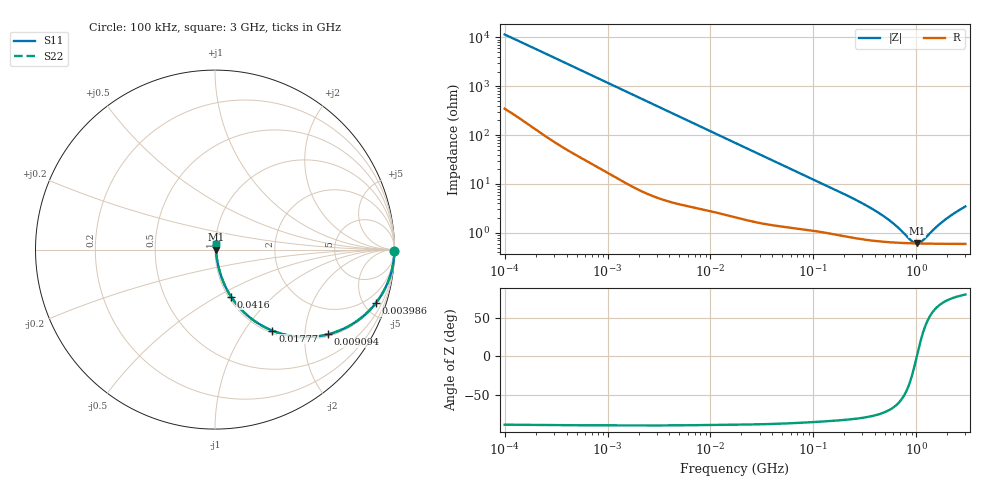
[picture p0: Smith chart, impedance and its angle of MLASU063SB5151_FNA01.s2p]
! MLASU063SB5151_FNA01  S-PARAMETER MODEL  ( Standard Model )
! Model Generated by TAIYO YUDEN Corporation (http://www.ty-top.com)
! Version 1.0
! TAIYO YUDEN Control No. 220601
! Copyright(c) 2012 TAIYO YUDEN CO.,LTD. All Rights Reserved.
! Product Description (link to TY-COMPAS)
! https://ds.yuden.co.jp/TYCOMPAS/or/detail?pn=MLASU063SB5151KFNA01&u=M
! Products Name : Multilayer Ceramic Capacitors
! Characteristics :
!  Capacitance : 150 [pF] , Rated Voltage : 50 [V] , TCC : B / X5R
!  Case Size : 0.6 x 0.3 / 0.024 x 0.012 [mm/inch] , Thickness : 0.3 / 0.012 [mm/inch]
!  (Conditions: Temperature = 25 [degC] , DC Bias Voltage = 0 [V])
! External Node Assignments :
!  1  o---| |---o  2
! GND o---------o GND
! Frequency Range : 100kHz  -  3GHz  [ 401 STEP ]
# MHZ S RI R 50
! Freq[MHz].  S11 Real  S11 Imag  S21 Real  S21 Imag  S12 Real  S12 Imag  S22 Real  S22 Imag
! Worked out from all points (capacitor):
!   401 points, 100 kHz to 3 GHz, reference 50 ohm
!   read as one part in series: C = 138 pF near 105.3 kHz
!   lowest |Z| = 606 mohm at 1.016 GHz (marker M1)
!   series resonance near 1.012 GHz, so ESL is about 180 pH
!   S11 on the Smith chart (normalised r, x): 100 kHz: open; 3.986 MHz: 1.09, -5.96; 9.094 MHz: 1.06, -2.63; 17.77 MHz: 1.04, -1.36; 41.6 MHz: 1.03, -0.58; 3 GHz: 1.01, +0.07
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0.1  0.9997 -0.00871  0.000339 0.00871  0.000339 0.00871  0.9997 -0.00871
0.562235  0.9969 -0.0477  0.00305 0.0477  0.00305 0.0477  0.9969 -0.0477
1.458987  0.9834 -0.1211  0.0166 0.1211  0.0166 0.1211  0.9834 -0.1211
3.161081  0.9309 -0.247  0.0691 0.247  0.0691 0.247  0.9309 -0.247
3.986308  0.8954 -0.2989  0.1046 0.2989  0.1046 0.2989  0.8954 -0.2989
6.020821  0.7924 -0.3969  0.2076 0.3969  0.2076 0.3969  0.7924 -0.3969
9.093698  0.6308 -0.4717  0.3692 0.4717  0.3692 0.4717  0.6308 -0.4717
12.71297  0.4721 -0.4864  0.5279 0.4864  0.5279 0.4864  0.4721 -0.4864
17.7727  0.3202 -0.4517  0.6798 0.4517  0.6798 0.4517  0.3202 -0.4517
26.84345  0.1781 -0.3646  0.8219 0.3646  0.8219 0.3646  0.1781 -0.3646
41.60216  0.0896 -0.2624  0.9104 0.2624  0.9104 0.2624  0.0896 -0.2624
97.38194  0.0262 -0.1217  0.9738 0.1217  0.9738 0.1217  0.0262 -0.1217
287.4592  0.00907 -0.0406  0.9909 0.0406  0.9909 0.0406  0.00907 -0.0406
412.3589  0.00739 -0.026  0.9926 0.026  0.9926 0.026  0.00739 -0.026
547.5153  0.00665 -0.0167  0.9933 0.0167  0.9933 0.0167  0.00665 -0.0167
672.8816  0.00632 -0.0107  0.9937 0.0107  0.9937 0.0107  0.00632 -0.0107
893.4279  0.00608 -0.00319  0.9939 0.00319  0.9939 0.00319  0.00608 -0.00319
1016.304  0.00602 0.00012  0.994 -0.00012  0.994 -0.00012  0.00602 0.00012
1156.079  0.006 0.00344  0.994 -0.00344  0.994 -0.00344  0.006 0.00344
1575.075  0.00607 0.0117  0.9939 -0.0117  0.9939 -0.0117  0.00607 0.0117
1935.725  0.00623 0.0179  0.9938 -0.0179  0.9938 -0.0179  0.00623 0.0179
3000  0.00703 0.0337  0.993 -0.0337  0.993 -0.0337  0.00703 0.0337
